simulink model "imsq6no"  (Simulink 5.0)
settings: Solver=ode45  StartTime=0  StopTime=0.02  MaxStep=4e-5  RelTol=1e-3  AbsTol=1e-3
InitFcn:
  | ic=[0.8330    0.0029   -0.9467    0.0026   -0.9784];
undefined symbols (not defined in the file or in its folder): sgn
libraries: simulink x1, mrlib x1

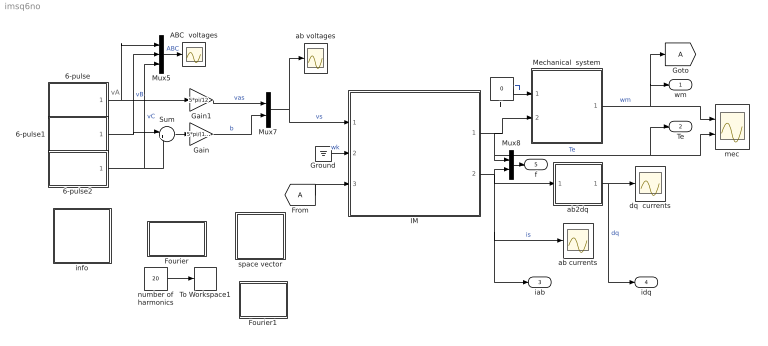
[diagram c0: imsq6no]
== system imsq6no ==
  note: vA
  6-pulse : Subsystem  mask{A=1, w=2*pi*50, p=1e-3}
      mask prompts: A "Amplitude"; w "Frequency [rad/s]"; p "Phase [rad]"
  6-pulse1 : Subsystem  mask{A=1.0, w=2*pi*50, p=-2*pi/3+1e-3}
      mask prompts: A "Amplitude"; w "Frequency [rad/s]"; p "Phase [rad]"
  6-pulse2 : Subsystem  mask{A=1.0, w=2*pi*50, p=2*pi/3+1e-3}
      mask prompts: A "Amplitude"; w "Frequency [rad/s]"; p "Phase [rad]"
  ABC  voltages : Scope
  Fourier : Subsystem
  Fourier1 : Subsystem
  Gain : Gain  Gain=5*pi/(12*sqrt(3))
  Gain1 : Gain  Gain=5*pi/12
  Ground : Ground
  IM : Subsystem  mask{Rs=0.01, Rr=0.02, Lsl=0.10, Lrl=0.10, Lm=4.5, wo=2*pi*60}
      mask prompts: Rs "Stator resistance [pu]"; Rr "Rotor resistance [pu]"; Lsl "Stator leakage inductance [pu]"; Lrl "Rotor leakage inductance [pu]"; Lm "Magnetizing inductance [pu]"; wo "Base frequency [rad/s]"
  Mechanical  system : Subsystem  mask{H=0.3, Bm=1e-5}
      mask prompts: H "Inertia constant [s]"; Bm "Torque-speed coefficient"
  Mux5 : Mux  Inputs=3
  Mux7 : Mux  Inputs=2
  Mux8 : Mux  Inputs=2
  Sum : Sum  Inputs=|+-
  Tl : Constant  Value=0
  To Workspace1 : ToWorkspace  VariableName=h  SampleTime=-1  SaveFormat=Array
  ab currents : Scope
  ab voltages : Scope
  ab2dq : Subsystem
  dq  currents : Scope
  info : Subsystem
  mec : Scope  NumInputPorts=2
  number of harmonics : Constant  Value=20
  space vector : Subsystem
  wm : Outport
  Te : Outport  Port=2
  iab : Outport  Port=3
  idq : Outport  Port=4
  f : Outport  Port=5
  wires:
  Sum/1 -> Gain/1
  6-pulse1/1(Out1) -> Sum/1, Mux5/2  "vB"
  6-pulse2/1(Out1) -> Sum/2, Mux5/3  "vC"
  6-pulse/1(Out1) -> Mux5/1, Gain1/1
  Mux5/1 -> ABC  voltages/1  "ABC"
  Gain/1 -> Mux7/2  "b"
  Gain1/1 -> Mux7/1  "vas"
  Mux7/1 -> ab voltages/1, IM/1(vs)  "vs"
  Ground/1 -> IM/2(wk)  "wk"
  Tl/1 -> Mechanical  system/1(Tl)  "Tl"
  Mechanical  system/1(wm) -> mec/1, wm/1, [A]  "wm"
  IM/1(Te) -> Mechanical  system/2(Te), mec/2, Te/1, Mux8/1  "Te"
  [A] -> IM/3(wm)
  ab2dq/1(dq) -> dq  currents/1, idq/1  "dq"
  Mux8/1 -> f/1
  IM/2(is) -> ab2dq/1(ab), ab currents/1, iab/1, Mux8/2  "is"
  number of harmonics/1 -> To Workspace1/1

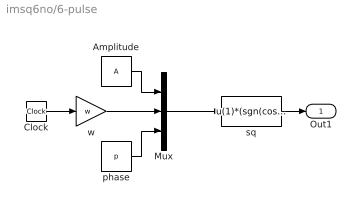
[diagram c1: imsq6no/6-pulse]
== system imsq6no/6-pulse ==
  Amplitude : Constant  Value=A
  Clock : Clock
  Mux : Mux  Inputs=3
  phase : Constant  Value=p
  sq : Fcn  Expr=u(1)*(sgn(cos(u(2)+u(3)))/2+sgn(cos(-3*(u(2)+u(3))))/6)
  w : Gain  Gain=w
  Out1 : Outport
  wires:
  Mux/1 -> sq/1
  sq/1 -> Out1/1
  Clock/1 -> w/1
  w/1 -> Mux/2
  phase/1 -> Mux/3
  Amplitude/1 -> Mux/1

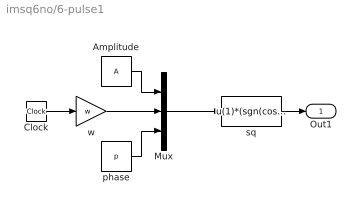
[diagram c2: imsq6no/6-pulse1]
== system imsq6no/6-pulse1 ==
  Amplitude : Constant  Value=A
  Clock : Clock
  Mux : Mux  Inputs=3
  phase : Constant  Value=p
  sq : Fcn  Expr=u(1)*(sgn(cos(u(2)+u(3)))/2+sgn(cos(-3*(u(2)+u(3))))/6)
  w : Gain  Gain=w
  Out1 : Outport
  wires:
  Amplitude/1 -> Mux/1
  phase/1 -> Mux/3
  w/1 -> Mux/2
  Clock/1 -> w/1
  sq/1 -> Out1/1
  Mux/1 -> sq/1

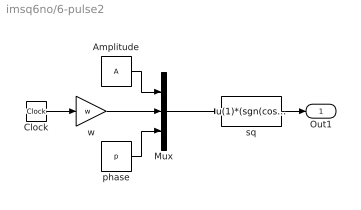
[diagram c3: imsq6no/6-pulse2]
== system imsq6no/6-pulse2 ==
  Amplitude : Constant  Value=A
  Clock : Clock
  Mux : Mux  Inputs=3
  phase : Constant  Value=p
  sq : Fcn  Expr=u(1)*(sgn(cos(u(2)+u(3)))/2+sgn(cos(-3*(u(2)+u(3))))/6)
  w : Gain  Gain=w
  Out1 : Outport
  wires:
  Mux/1 -> sq/1
  sq/1 -> Out1/1
  Clock/1 -> w/1
  w/1 -> Mux/2
  phase/1 -> Mux/3
  Amplitude/1 -> Mux/1

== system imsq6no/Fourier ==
  note: To obtain the Fourier decomposition of a periodic signal: a) run a simulation for one period duration b) Specify the fundamental frequency c) Specify the number of harmonics

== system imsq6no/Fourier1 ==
  note: To obtain the Fourier decomposition of a periodic signal: a) run a simulation for one period duration b) Specify the fundamental frequency c) Specify the number of harmonics

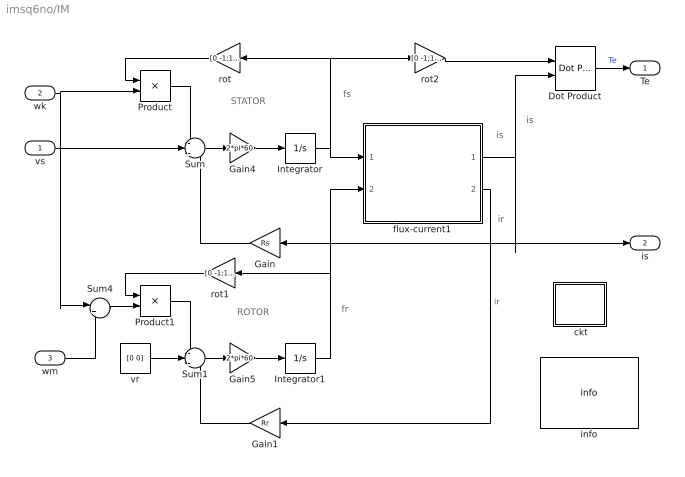
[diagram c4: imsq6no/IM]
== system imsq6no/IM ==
  note: ROTOR
  note: STATOR
  note: fs
  note: fr
  note: is
  note: is
  note: ir
  vs : Inport
  wk : Inport  Port=2
  wm : Inport  Port=3
  " ckt" : Subsystem
  Dot Product : simulink/Math Operations/Dot Product
  Gain : Gain  Orientation=left  Gain=Rs
  Gain1 : Gain  Orientation=left  Gain=Rr
  Gain4 : Gain  Gain=2*pi*60
  Gain5 : Gain  Gain=2*pi*60
  Integrator : Integrator  InitialCondition=[0 0]
  Integrator1 : Integrator  InitialCondition=[0 0]
  Product : Product
  Product1 : Product
  Sum : Sum  Inputs=-+-
  Sum1 : Sum  Inputs=-+-
  Sum4 : Sum  Inputs=|+-
  flux-current1 : Subsystem
  info : mrlib/IM/info
  rot : Gain  Orientation=left  Gain=[0 -1;1 0]  Multiplication=Matrix(K*u)
  rot1 : Gain  Orientation=left  Gain=[0 -1;1 0]  Multiplication=Matrix(K*u)
  rot2 : Gain  Gain=[0 -1;1 0]  Multiplication=Matrix(K*u)
  vr : Constant  Value=[0 0]
  Te : Outport
  is : Outport  Port=2
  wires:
  Gain/1 -> Sum/3
  vr/1 -> Sum1/2
  Gain1/1 -> Sum1/3
  flux-current1/2(ir) -> Gain1/1  "ir"
  Integrator/1 -> flux-current1/1(fs), rot/1, rot2/1
  Integrator1/1 -> flux-current1/2(fr), rot1/1
  Product1/1 -> Sum1/1
  rot1/1 -> Product1/1
  Product/1 -> Sum/1
  rot/1 -> Product/1
  rot2/1 -> Dot Product/1
  Sum4/1 -> Product1/2
  Sum/1 -> Gain4/1
  Gain4/1 -> Integrator/1
  Sum1/1 -> Gain5/1
  Gain5/1 -> Integrator1/1
  flux-current1/1(is) -> Gain/1, is/1, Dot Product/2
  Dot Product/1 -> Te/1  "Te"
  vs/1 -> Sum/2
  wk/1 -> Product/2, Sum4/1
  wm/1 -> Sum4/2

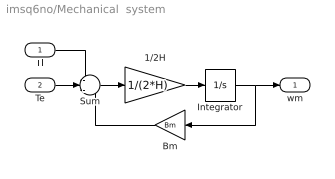
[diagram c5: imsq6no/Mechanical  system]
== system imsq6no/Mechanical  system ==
  Tl : Inport
  Te : Inport  Port=2
  1/2H : Gain  Gain=1/(2*H)
  Bm : Gain  Orientation=left  Gain=Bm
  Integrator : Integrator  InitialCondition=.82
  Sum : Sum  Inputs=-+-
  wm : Outport
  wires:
  Tl/1 -> Sum/1
  Te/1 -> Sum/2
  Integrator/1 -> wm/1, Bm/1
  Bm/1 -> Sum/3
  Sum/1 -> 1/2H/1
  1/2H/1 -> Integrator/1

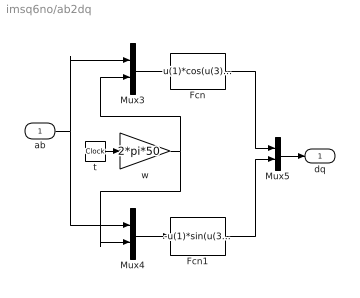
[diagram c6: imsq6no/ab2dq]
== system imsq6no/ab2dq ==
  ab : Inport
  Fcn : Fcn  Expr=u(1)*cos(u(3))+u(2)*sin(u(3))
  Fcn1 : Fcn  Expr=-u(1)*sin(u(3))+u(2)*cos(u(3))
  Mux3 : Mux  Inputs=2
  Mux4 : Mux  Inputs=2
  Mux5 : Mux  Inputs=2
  t : Clock
  w : Gain  Gain=2*pi*50
  dq : Outport
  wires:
  t/1 -> w/1
  Mux3/1 -> Fcn/1
  Mux4/1 -> Fcn1/1
  w/1 -> Mux3/2, Mux4/2
  ab/1 -> Mux3/1, Mux4/1
  Fcn1/1 -> Mux5/2
  Fcn/1 -> Mux5/1
  Mux5/1 -> dq/1

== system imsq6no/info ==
  note: An induction motor under 6-pulse squarewave excitation
  note: This model shows the steady-state conditions of the motor when it operates at no load

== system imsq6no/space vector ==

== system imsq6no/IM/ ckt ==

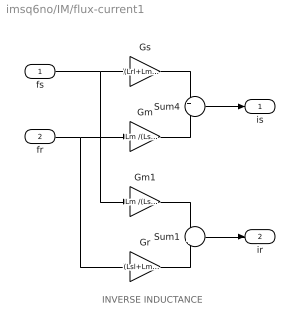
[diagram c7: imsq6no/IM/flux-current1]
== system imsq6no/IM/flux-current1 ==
  note: INVERSE INDUCTANCE
  fs : Inport
  fr : Inport  Port=2
  Gm : Gain  Gain=Lm /(Lsl*Lrl+Lsl*Lm+Lrl*Lm)
  Gm1 : Gain  Gain=Lm /(Lsl*Lrl+Lsl*Lm+Lrl*Lm)
  Gr : Gain  Gain=(Lsl+Lm )/(Lsl*Lrl+Lsl*Lm+Lrl*Lm)
  Gs : Gain  Gain=(Lrl+Lm) /(Lsl*Lrl+Lsl*Lm+Lrl*Lm)
  Sum1 : Sum  Inputs=-+
  Sum4 : Sum  Inputs=+-
  is : Outport
  ir : Outport  Port=2
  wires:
  fs/1 -> Gs/1, Gm1/1
  Gs/1 -> Sum4/1
  fr/1 -> Gm/1, Gr/1
  Gm/1 -> Sum4/2
  Sum4/1 -> is/1
  Gm1/1 -> Sum1/1
  Gr/1 -> Sum1/2
  Sum1/1 -> ir/1
